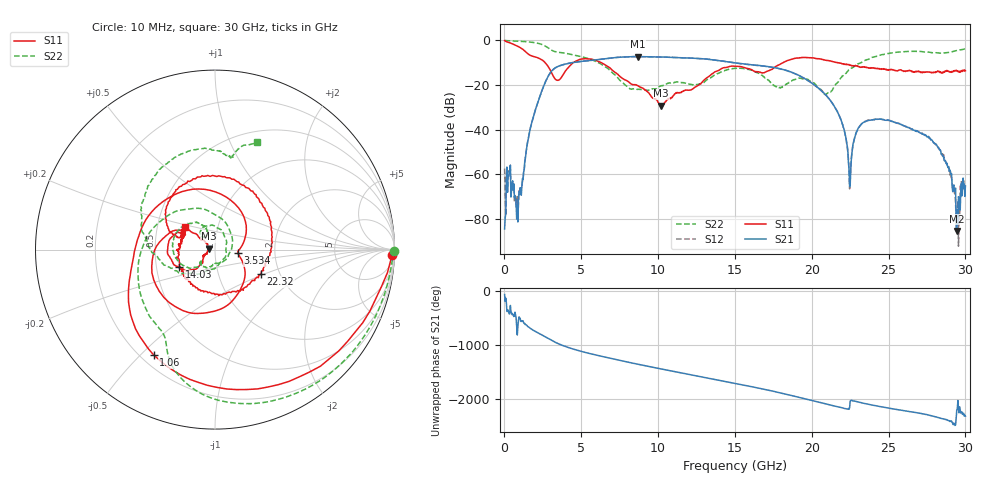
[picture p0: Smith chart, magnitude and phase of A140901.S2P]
!  2-Port S-parameters saved by WinCal
! VAR MeasName=S-Parameters (CALIBRATED_DATA) read from VNA (N5244A)
! VAR MeasDate=11/3/2014 9:26:24 AM
! VAR NAME=A140901
! VAR FILENAME=A140901.S2P
! VAR DATE=11/3/2014 9:26:24 AM
! VAR PHYS_PORTS=1,2
# Hz S RI R 50
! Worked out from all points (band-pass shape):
!   801 points, 10 MHz to 30 GHz, reference 50 ohm
!   highest |S21| = -7.24 dB at 8.67 GHz (marker M1); lowest = -85.2 dB at 29.44 GHz (marker M2)
!   |S21| within 3 dB of the highest: 4.194 GHz to 15.2 GHz (11.01 GHz wide, 114 % of centre)
!   lowest |S11| = -29.2 dB at 10.21 GHz (marker M3), VSWR 1.07, Z = 46.7 + j0.409 ohm
!   |S11| at or under -10 dB: 2.65 GHz to 4.471 GHz (1.821 GHz wide, 51.1 % of centre); 6.307 GHz to 18.13 GHz (11.83 GHz wide, 96.8 % of centre); 21.67 GHz to end of sweep
!   |S22| runs from -24.4 to 0.0 dB; largest |S21 - S12| = 0.0034
!   S11 on the Smith chart (normalised r, x): 10 MHz: 22, -53; 1.06 GHz: 0.25, -0.55; 3.534 GHz: 1.29, -0.05; 14.03 GHz: 0.66, -0.14; 22.32 GHz: 1.60, -0.48; 30 GHz: 0.70, +0.18
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1e7  0.9863 -0.0319  1.91e-05 -5.71e-05  8.65e-05 0.00135  0.9951 -0.00843
2.724125e8  0.7397 -0.5101  0.000639 -0.000642  0.000862 -0.000844  0.9642 -0.1776
7.972375e8  -0.0409 -0.7565  5.54e-05 8.38e-05  -1.53e-06 0.000161  0.8377 -0.4731
1.05965e9  -0.3423 -0.5866  -0.000326 0.000169  -0.000251 0.000224  0.7394 -0.5982
2.071812e9  -0.3853 0.1663  0.0228 -0.0228  0.0227 -0.0229  0.1714 -0.8579
3.533825e9  0.1279 -0.0203  -0.0205 0.2648  -0.0209 0.2647  -0.3044 -0.4453
5.033325e9  -0.1785 -0.34  0.2312 -0.2477  0.2311 -0.2482  -0.4249 -0.0649
6.982675e9  -0.1932 0.1083  -0.4051 -0.0117  -0.4053 -0.0117  0.00265 0.1927
8.669612e9  -0.0791 0.0562  0.0917 0.4245  0.0919 0.4242  0.0458 -0.0655
1.001916e10  -0.0394 0.011  0.4251 0.000264  0.4245 -3.46e-05  -0.0156 -0.0891
1.02066e10  -0.0342 0.00438  0.4164 -0.0779  0.415 -0.0775  -0.0206 -0.0933
1.181856e10  -0.0658 -0.04  -0.0738 -0.398  -0.075 -0.3984  -0.0828 -0.07
1.403032e10  -0.2002 -0.0987  -0.2457 0.2494  -0.245 0.2494  -0.1684 -0.0918
1.5005e10  -0.2633 0.0121  0.0493 0.31  0.0513 0.3081  -0.2352 0.0138
1.766661e10  -0.2438 0.0964  0.0671 -0.2328  0.0669 -0.2327  -0.0421 0.0811
2.002832e10  0.083 0.3997  -0.0618 0.0899  -0.0625 0.089  0.0305 0.1124
2.167778e10  0.3141 0.0293  0.0247 0.00382  0.0246 0.00408  -0.0199 -0.1122
2.231506e10  0.2566 -0.136  0.00355 -0.00225  0.00349 -0.00225  -0.1469 -0.1324
2.501416e10  -0.1839 -0.1131  0.0156 -0.00436  0.0157 -0.00426  -0.3748 0.3488
2.82006e10  -0.1909 0.0812  -0.00408 0.000603  -0.00394 0.000487  0.08 0.5192
2.943769e10  -0.1853 0.1014  3.23e-05 -4.42e-05  0.000141 4.13e-05  0.149 0.5758
3e10  -0.1659 0.1272  -0.000533 -0.000155  -0.000559 -9.6e-05  0.2339 0.5985
